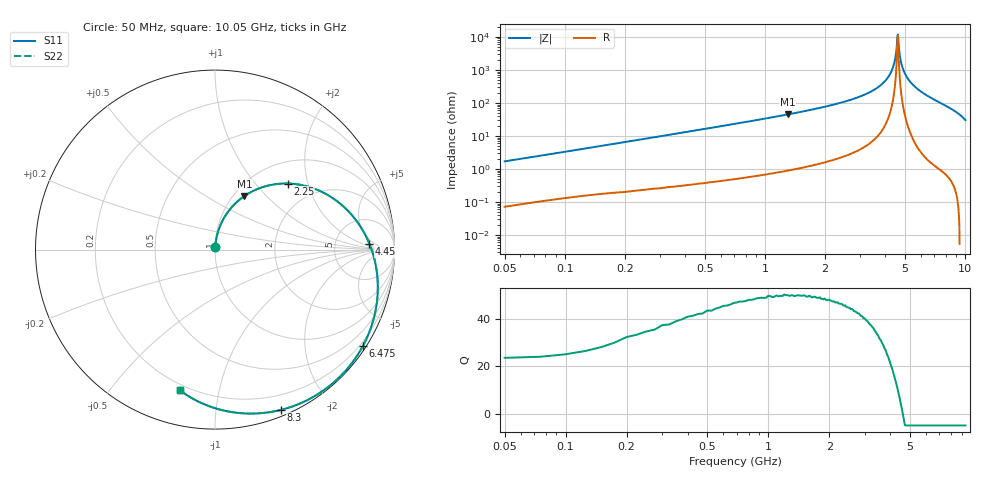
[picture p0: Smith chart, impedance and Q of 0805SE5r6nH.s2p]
! AVX Thin Film Operation		Date: May 2002
! Description: Accu-L® Series, Thin Film, SMD, RF Inductors
! Part Number: L08055R6CEWTR
! 50 MHz  -  10.05 GHz
! Serial Measurements
# mhz S db R 50
!	S11		S21		S12		S22
!	dB	Phase	dB	Phase	dB	Phase	dB	Phase
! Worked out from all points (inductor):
!   401 points, 50 MHz to 10.05 GHz, reference 50 ohm
!   read as 1/Y11, port 2 shorted: L = 5.27 nH near 100 MHz
!   highest Q = 50.1 at 1.3 GHz (marker M1), where L = 5.52 nH
!   self-resonance near 4.6 GHz
!   S11 on the Smith chart (normalised r, x): 50 MHz: 1.00, +0.03; 2.25 GHz: 1.43, +1.50; 4.45 GHz: 13, +3; 6.475 GHz: 0.10, -3.35; 8.3 GHz: 0.06, -1.49; 10.05 GHz: 0.17, -0.77
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50  -36.64 85.9  -0.01 -1.1  -0.01 -1.1  -36.64 85.9
200  -25.03 83.6  -0.03 -4.3  -0.03 -4.3  -25.03 83.6
425  -18.63 79.2  -0.09 -9.1  -0.09 -9.1  -18.63 79.2
775  -13.58 72.0  -0.23 -16.4  -0.23 -16.4  -13.58 72.0
1300  -9.35 61.2  -0.59 -27.1  -0.59 -27.1  -9.35 61.2
1725  -7.16 52.6  -0.99 -35.6  -0.99 -35.6  -7.16 52.6
2250  -5.23 42.3  -1.63 -45.7  -1.63 -45.7  -5.23 42.3
3400  -2.63 20.7  -3.56 -66.7  -3.56 -66.7  -2.63 20.7
4450  -1.30 2.1  -6.11 -84.7  -6.11 -84.7  -1.30 2.1
5050  -0.80 -8.3  -8.10 -94.7  -8.10 -94.7  -0.80 -8.3
5900  -0.33 -23.0  -12.27 -108.5  -12.27 -108.5  -0.33 -23.0
6475  -0.14 -33.2  -17.25 -117.4  -17.25 -117.4  -0.14 -33.2
6725  -0.10 -37.7  -20.93 -120.4  -20.93 -120.4  -0.10 -37.7
6975  -0.07 -42.3  -27.59 -120.2  -27.59 -120.2  -0.07 -42.3
7150  -0.06 -45.5  -38.20 -64.4  -38.20 -64.4  -0.06 -45.5
7200  -0.06 -46.4  -43.47 -17.5  -43.47 -17.5  -0.06 -46.4
7375  -0.07 -49.7  -28.36 34.1  -28.36 34.1  -0.07 -49.7
7550  -0.09 -53.0  -22.73 35.8  -22.73 35.8  -0.09 -53.0
7850  -0.15 -58.7  -17.46 32.4  -17.46 32.4  -0.15 -58.7
8300  -0.30 -67.6  -12.90 24.7  -12.90 24.7  -0.30 -67.6
8400  -0.35 -69.6  -12.14 22.8  -12.14 22.8  -0.35 -69.6
10050  -1.84 -103.9  -4.87 -10.9  -4.87 -10.9  -1.84 -103.9
